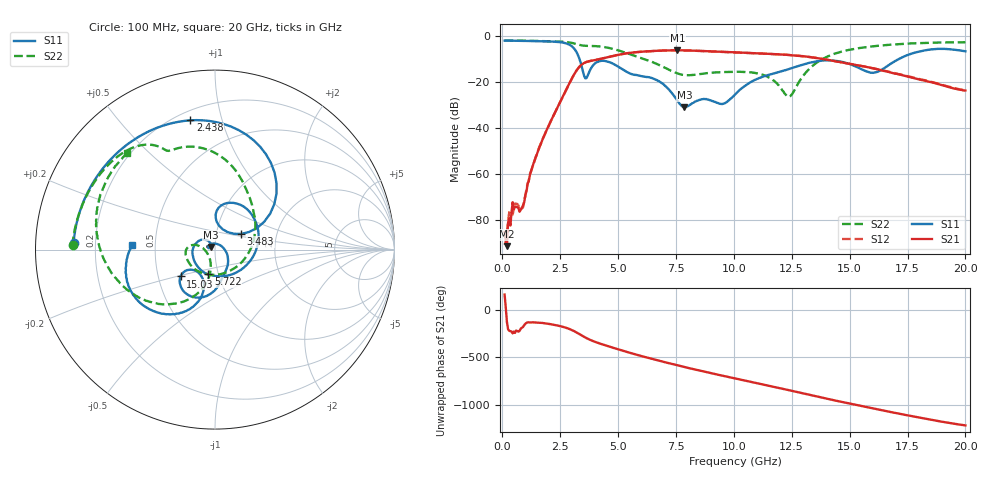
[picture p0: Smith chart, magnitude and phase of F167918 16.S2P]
!  2-Port S-parameters saved by WinCal
! VAR MeasName=S-Parameters (CALIBRATED_DATA) read from VNA (N5242A)
! VAR MeasDate=2016-11-22 10:25:33
! VAR NAME=F167918 16
! VAR FILENAME=F167918 16.S2P
! VAR DATE=2016-11-22 10:25:33
! VAR PHYS_PORTS=1,2
# Hz S DB R 50
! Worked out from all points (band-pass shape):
!   401 points, 100 MHz to 20 GHz, reference 50 ohm
!   highest |S21| = -6.27 dB at 7.562 GHz (marker M1); lowest = -91.2 dB at 199.5 MHz (marker M2)
!   |S21| within 3 dB of the highest: 4.55 GHz to 13.32 GHz (8.769 GHz wide, 98.2 % of centre)
!   lowest |S11| = -31.0 dB at 7.861 GHz (marker M3), VSWR 1.06, Z = 47.6 + j1.37 ohm
!   |S11| at or under -10 dB: 3.332 GHz to 17.14 GHz (13.81 GHz wide, 135 % of centre)
!   |S22| runs from -26.5 to -2.0 dB; largest |S21 - S12| = 0.0041
!   S11 on the Smith chart (normalised r, x): 100 MHz: 0.12, +0.02; 2.438 GHz: 0.25, +0.79; 3.483 GHz: 1.32, +0.24; 5.722 GHz: 0.89, -0.25; 15.03 GHz: 0.65, -0.21; 20 GHz: 0.37, +0.02
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1e8  -2.07 177.3  -85.09 159.7  -90.63 136.0  -2.00 178.3
1.995e8  -2.08 174.6  -91.23 -128.1  -85.44 94.5  -2.01 176.6
8.4625e8  -2.18 157.3  -74.45 170.7  -74.87 176.1  -2.11 166.1
1.493e9  -2.29 138.5  -51.44 -133.6  -51.18 -134.2  -2.22 155.5
2.43825e9  -2.69 100.9  -29.93 -168.6  -29.90 -169.2  -2.46 137.6
3.085e9  -5.31 52.3  -17.02 137.2  -17.04 136.9  -3.24 121.9
3.43325e9  -13.43 27.3  -12.44 88.8  -12.43 88.7  -4.13 116.5
3.483e9  -15.41 31.0  -12.09 81.9  -12.07 81.7  -4.22 116.1
4.52775e9  -11.12 38.3  -9.32 -19.8  -9.34 -20.1  -5.09 93.8
5.72175e9  -16.94 -105.2  -7.12 -107.4  -7.11 -107.4  -8.68 60.7
6.7665e9  -19.69 152.7  -6.44 -175.3  -6.45 -175.5  -12.61 19.6
7.5625e9  -28.12 128.0  -6.27 136.1  -6.30 136.0  -16.27 -38.2
7.861e9  -30.97 149.4  -6.32 118.3  -6.32 118.3  -17.01 -65.3
8.80625e9  -27.40 146.6  -6.65 65.1  -6.65 64.9  -16.21 -131.0
1.005e10  -25.47 1.1  -7.14 -1.6  -7.16 -1.5  -15.62 -167.4
1.13435e10  -17.43 -64.6  -7.72 -69.8  -7.71 -69.4  -17.21 170.4
1.238825e10  -14.37 -82.5  -8.31 -125.7  -8.27 -125.7  -26.46 -147.4
1.338325e10  -11.43 -102.4  -9.34 179.2  -9.29 179.4  -13.18 -107.1
1.5025e10  -12.30 -142.0  -12.22 93.1  -12.15 93.1  -5.99 -147.9
1.67165e10  -12.54 -105.6  -15.69 7.8  -15.64 8.3  -3.89 179.9
1.815925e10  -6.45 -132.5  -19.25 -59.6  -19.05 -59.8  -3.08 157.4
2e10  -6.70 177.0  -23.72 -135.9  -23.63 -136.6  -2.78 132.5
